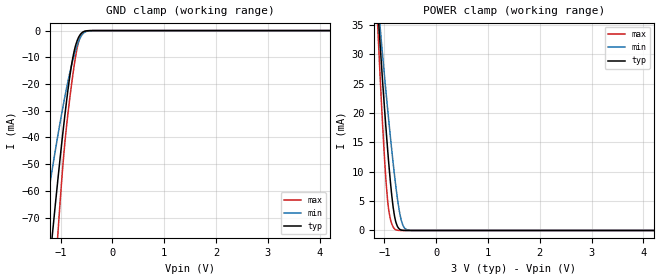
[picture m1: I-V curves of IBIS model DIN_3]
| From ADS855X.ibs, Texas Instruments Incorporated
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|   INPUT 3.0V model
[Model]   DIN_3
Model_type   Input
| Signals   CS/FS, RD, CONVST_C, CONVST_B, CONVST_A, STBY, RANGE/XCLK,
|   RESET, WORD/BYTE, PAR/SER, HW/SW,REFEN/WR
Vinl = -300.000mV   |min, BGND -0.3V
Vinh = 3.6V   |max. BVDD +0.3V
| C_comp   obtained at 25MHz
| variable   typ   min   max
C_comp   3.806pF   2.861pF   4.719pF
[Temperature Range]   40.0   125.0   -40.0
[Voltage range]   3.0V   2.7V   3.3V
[power clamp reference] 3.0V   2.7V   3.3V
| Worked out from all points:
|   GND clamp passes 1 mA (typ) near -0.60 V on its own axis
|   POWER clamp passes 1 mA (typ) near -0.76 V on its own axis
[GND Clamp]
|   Voltage   I(typ)   I(min)   I(max)
-3V       -493.1mA   -328.5mA   -702.2mA
-1.383V   -122.5mA   -79.89mA   -177.4mA
-1.326V   -110.4mA   -72.39mA   -159.3mA
-1.179V   -80.14mA   -53.91mA   -113.4mA
-1.121V   -68.8mA    -47.05mA   -96.04mA
-1.054V   -55.86mA   -39.26mA   -76.29mA
-917.6mV  -31.58mA   -24.69mA   -41.86mA
-787.1mV  -12.59mA   -12.82mA   -19.83mA
-721.9mV  -6.351mA   -8.03mA    -10.97mA
-660mV    -2.796mA   -4.418mA   -4.757mA
-549.8mV  -340.5uA   -799.5uA   -408.9uA
5.999V    0A         0A         0A
[POWER Clamp]
|   Voltage   I(typ)   I(min)   I(max)
-3V       226.3mA    192mA      270.5mA
-1.136V   38.85mA    40.03mA    35.99mA
-1.107V   34.88mA    37.04mA    30.59mA
-1.072V   30.23mA    33.52mA    24.33mA
-996.4mV  20.62mA    26.16mA    12.09mA
-939mV    13.94mA    20.82mA    5.225mA
-910.9mV  10.94mA    18.28mA    3.164mA
-845.6mV  5.024mA    12.67mA    875.5uA
-773.6mV  1.289mA    7.125mA    95.94uA
-656.6mV  44.02uA    1.217mA    1.965uA
-494.6mV  190nA      16.18uA    -23.79nA
5.999V    -35.58nA   -43.76nA   -28.45nA
